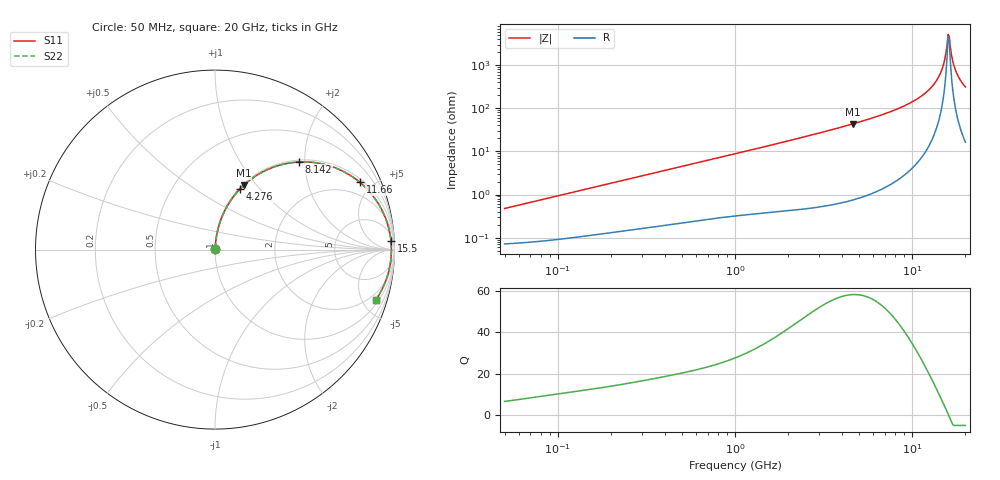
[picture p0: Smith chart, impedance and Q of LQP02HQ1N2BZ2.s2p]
!Murata Part Number: LQP02HQ1N2BZ2
!These Parameters are Measured in Series Mode Connection
!  o--[Z]--o
!Port1  Port2
!  o-------o
!Freq. Start=50[MHz] Stop=20[GHz], 401[Steps]
# Hz S RI R 50
!Freq.(Hz) S11(Real) S11(Imag) S21(Real) S21(Imag) S12(Real) S12(Imag) S22(Real) S22(Imag)
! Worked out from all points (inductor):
!   401 points, 50 MHz to 20 GHz, reference 50 ohm
!   read as one part in series: L = 1.49 nH near 51.52 MHz
!   highest Q = 58.1 at 4.608 GHz (marker M1), where L = 1.49 nH
!   self-resonance near 15.98 GHz
!   S11 on the Smith chart (normalised r, x): 50 MHz: 1.00, +0.01; 4.276 GHz: 1.01, +0.79; 8.142 GHz: 1.04, +1.88; 11.66 GHz: 1.17, +4.22; 15.5 GHz: 13, +34; 20 GHz: 1.33, -6.24
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5e7  0.000737 0.00469  0.9993 -0.00469  0.9993 -0.00469  0.000737 0.00469
1.364002e8  0.00122 0.0125  0.9988 -0.0125  0.9988 -0.0125  0.00122 0.0125
3.721004e8  0.00294 0.0331  0.9971 -0.0331  0.9971 -0.0331  0.00294 0.0331
1e9  0.0107 0.0862  0.9893 -0.0862  0.9893 -0.0862  0.0107 0.0862
2.728004e9  0.0593 0.2263  0.9407 -0.2263  0.9407 -0.2263  0.0593 0.2263
4.275624e9  0.1394 0.3378  0.8606 -0.3378  0.8606 -0.3378  0.1394 0.3378
4.608136e9  0.1611 0.3591  0.8389 -0.3591  0.8389 -0.3591  0.1611 0.3591
7.442007e9  0.4 0.4799  0.6 -0.4799  0.6 -0.4799  0.4 0.4799
8.141811e9  0.4697 0.4882  0.5303 -0.4882  0.5303 -0.4882  0.4697 0.4882
9.892087e9  0.6472 0.4639  0.3528 -0.4639  0.3528 -0.4639  0.6472 0.4639
1.166392e10  0.8074 0.3745  0.1926 -0.3745  0.1926 -0.3745  0.8074 0.3745
1.295331e10  0.896 0.2773  0.104 -0.2773  0.104 -0.2773  0.896 0.2773
1.417136e10  0.9516 0.171  0.0484 -0.171  0.0484 -0.171  0.9516 0.171
1.504638e10  0.974 0.0916  0.026 -0.0916  0.026 -0.0916  0.974 0.0916
1.550395e10  0.9802 0.0503  0.0198 -0.0503  0.0198 -0.0503  0.9802 0.0503
1.573793e10  0.9819 0.0294  0.0181 -0.0294  0.0181 -0.0294  0.9819 0.0294
1.621653e10  0.9828 -0.0125  0.0172 0.0125  0.0172 0.0125  0.9828 -0.0125
1.646126e10  0.9818 -0.0335  0.0182 0.0335  0.0182 0.0335  0.9818 -0.0335
1.721783e10  0.9737 -0.0957  0.0263 0.0957  0.0263 0.0957  0.9737 -0.0957
1.774144e10  0.964 -0.136  0.036 0.136  0.036 0.136  0.964 -0.136
1.88369e10  0.9351 -0.2125  0.0649 0.2125  0.0649 0.2125  0.9351 -0.2125
2e10  0.8951 -0.2814  0.1049 0.2814  0.1049 0.2814  0.8951 -0.2814
